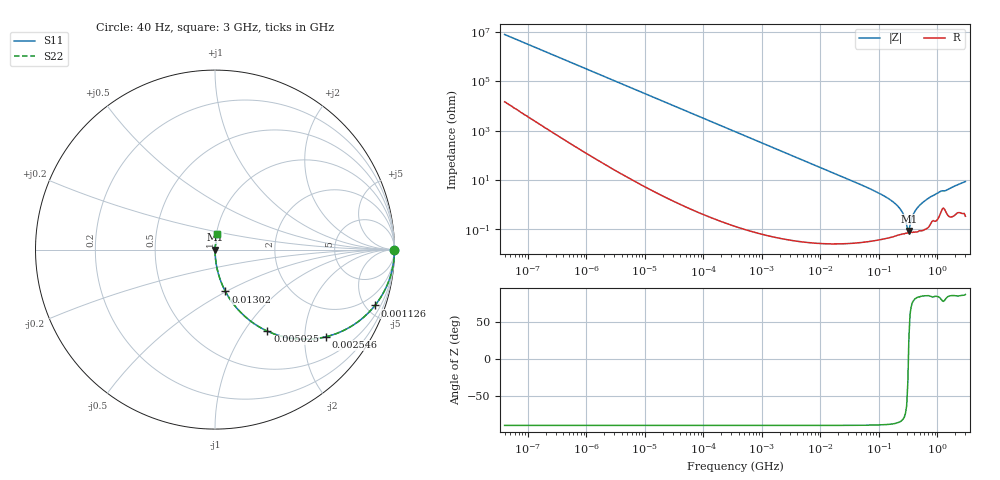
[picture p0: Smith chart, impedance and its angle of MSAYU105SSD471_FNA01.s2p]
! MSAYU105SSD471_FNA01  S-PARAMETER MODEL  ( General Type )
! Model Generated by TAIYO YUDEN Corporation (http://www.ty-top.com)
! Version 2.0
! TAIYO YUDEN Control No. 051115
! Copyright(c) 2005 TAIYO YUDEN CO.,LTD. All Rights Reserved.
! Product Description (link to TY-COMPAS)
! https://ds.yuden.co.jp/TYCOMPAS/or/detail?pn=MSAYU105SSD471KFNA01&u=M
! Products Name : Multilayer Ceramic Capacitors
! Characteristics :
!  Capacitance : 470 pF , Rated Voltage : 50V
!  Case Size : 1.0 x 0.5 / 0.039 x 0.02 [mm/inch] , Thickness : 0.5 / 0.02 [mm/inch]
!  (Conditions: Temperature = 25 degC , DC Bias Current/Voltage = 0A / 0V)
! External Node Assignments :
!  1  o---| |---o  2
! GND o---------o GND
! Frequency Range : 40Hz  -  3GHz  [ 401 STEP ]
# MHz S RI R 50
! Freq[MHz].  S11 Real  S11 Imag  S21 Real  S21 Imag  S12 Real  S12 Imag  S22 Real  S22 Imag
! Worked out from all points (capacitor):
!   401 points, 40 Hz to 3 GHz, reference 50 ohm
!   read as one part in series: C = 494 pF near 44 Hz
!   lowest |Z| = 85.4 mohm at 325.4 MHz (marker M1)
!   series resonance near 318.4 MHz, so ESL is about 510 pH
!   S11 on the Smith chart (normalised r, x): 40 Hz: open; 1.126 MHz: 1.00, -5.73; 2.546 MHz: 1.00, -2.53; 5.025 MHz: 1.00, -1.28; 13.02 MHz: 1.00, -0.49; 3 GHz: 1.01, +0.17
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4e-05  1 -1.24e-05  2.3e-08 1.24e-05  2.3e-08 1.24e-05  1 -1.24e-05
0.000308  1 -9.55e-05  7.1e-08 9.55e-05  7.1e-08 9.55e-05  1 -9.55e-05
0.000834  1 -0.000259  1.71e-07 0.000259  1.71e-07 0.000259  1 -0.000259
0.017386  1 -0.00539  2.99e-05 0.00539  2.99e-05 0.00539  1 -0.00539
0.362475  0.9875 -0.111  0.0125 0.111  0.0125 0.111  0.9875 -0.111
1.125822  0.8912 -0.3112  0.1088 0.3112  0.1088 0.3112  0.8912 -0.3112
2.545935  0.6158 -0.4863  0.3842 0.4863  0.3842 0.4863  0.6158 -0.4863
5.025302  0.2915 -0.4542  0.7085 0.4542  0.7085 0.4542  0.2915 -0.4542
7.222098  0.1661 -0.3719  0.8339 0.3719  0.8339 0.3719  0.1661 -0.3719
13.01976  0.0578 -0.2328  0.9422 0.2328  0.9422 0.2328  0.0578 -0.2328
66.58224  0.00245 -0.0462  0.9975 0.0462  0.9975 0.0462  0.00245 -0.0462
150.5692  0.00072 -0.0165  0.9993 0.0165  0.9993 0.0165  0.00072 -0.0165
226.4253  0.000642 -0.00697  0.9994 0.00697  0.9994 0.00697  0.000642 -0.00697
259.4108  0.000664 -0.00414  0.9993 0.00414  0.9993 0.00414  0.000664 -0.00414
297.2015  0.000685 -0.00137  0.9993 0.00137  0.9993 0.00137  0.000685 -0.00137
325.4065  0.000732 0.000438  0.9993 -0.000438  0.9993 -0.000438  0.000732 0.000438
340.4975  0.000731 0.00134  0.9993 -0.00134  0.9993 -0.00134  0.000731 0.00134
390.1008  0.000784 0.00412  0.9992 -0.00412  0.9992 -0.00412  0.000784 0.00412
427.1222  0.00081 0.00602  0.9992 -0.00602  0.9992 -0.00602  0.00081 0.00602
586.632  0.0011 0.0132  0.9989 -0.0132  0.9989 -0.0132  0.0011 0.0132
1057.561  0.00406 0.0312  0.9959 -0.0312  0.9959 -0.0312  0.00406 0.0312
3000  0.0106 0.0846  0.9894 -0.0846  0.9894 -0.0846  0.0106 0.0846
